[IBIS ver]   4.2
[File name]   msp432e411ytzad_212bga_v0p0.ibs
[File Rev]   v0p0
[Date]   Oct 10, 2017
[Source]   simulation
[Notes]   IBIS models for 212BGA package with updated GPIO models
[Disclaimer] Please be aware that in the absence of a written agreement,
   Texas Instruments (TI) assumes no liability for: 1) the
   accuracy of the IBIS models provided to your company, 2) the
   proper functioning of these IBIS models in your design or for
   any resulting applications, or; 3) infringement of patents,
   copyrights, or intellectual property rights resulting from
   your use of these IBIS models. TI provides IBIS models as a
   service to our customers and therefore reserves the right to
   limit distribution of the IBIS models.
   This preliminary model does not contain all of the possible pad
   models for each of the pad types.  The most commonly used modes
   have been provided and the next update will include all of the
   pad model combinations.
   The only missing models that needs to be highlighted are the
   model for the USB D+ and D- GPIOs and the Ethernet PHY.
   Currently only the USB functionality is provided on the D+ and
   D- pins.  Customers needing to model the PGIOs associated with
   these pins should check for a newer model.  The Ethernet pins
   are curently shown as NC.  Although models will be provided in
   a future release, the magnetics and connector should be palced
   as close as possible to the device for best performance.
[Copyright]   Property of Texas Instruments Incorporated. Unauthorized
   reproduction and/or distribution is strictly prohibited. This
   product is protected under copyright law and trade secret law
   as an unpublished work. Copyright (C) 2017, Texas Instruments
   Incorporated, all rights reserved. These commodities are under
   the U.S. Government distribution license control. As such,
   they are not to be re-exported without the prior approval of
   the U.S. Department of Commerce.
|   Component MSP432E411YTZAD
[Component]   MSP432E411YTZAD
[Manufacturer]   Texas Instruments Inc.
[Package]
| 212-pin BGA
| variable   typ   min   max
R_Pkg   1.91E-01   1.42E-01   3.53E-01
L_pkg   2.25E-09   1.34E-09   5.30E-09
C_pkg   5.40E-13   3.57E-13   1.22E-12
[Pin]   signal_name   model_name   R_pin   L_pin   C_pin
A1   GND   GND
A2   GND   GND
A4   PD4   GPIO12P   2.07E-01   2.54212E-09   4.28804E-13
A5   PE4   GPIO12P   2.01E-01   2.46532E-09   4.18963E-13
A7   PE6   GPIO12P   1.94E-01   2.38893E-09   4.10699E-13
A8   PP7   GPIO12P   1.96E-01   2.49906E-09   4.59589E-13
A10   PN4   GPIO12P   1.93E-01   2.41012E-09   3.56985E-13
A11   PN2   GPIO12P   1.94E-01   2.32364E-09   3.86379E-13
A13   PQ4   GPIO12P   2.11E-01   2.54553E-09   4.60355E-13
A14   PS3   GPIO12P   2.08E-01   2.42399E-09   4.21739E-13
A16   PB0   GPIO8P_5V   2.00E-01   3.23551E-09   6.06843E-13
A17   PB2   GPIO12P   2.14E-01   3.52368E-09   5.43338E-13
A18   GND   GND
A19   GND   GND
B1   GND   GND
B2   PD7   GPIO12P   1.72E-01   2.14055E-09   4.66734E-13
B3   PD6   GPIO12P   1.60E-01   1.98098E-09   4.32256E-13
B4   PD5   GPIO12P   2.13E-01   2.5073E-09   4.43666E-13
B5   PE5   GPIO12P   1.84E-01   2.03073E-09   4.37429E-13
B6   PB5   GPIO12P   1.58E-01   1.89444E-09   4.1673E-13
B7   PE7   GPIO12P   1.80E-01   1.97736E-09   4.23857E-13
B8   PP6   GPIO12P   1.90E-01   2.22432E-09   5.22651E-13
B9   PN5   GPIO12P   1.82E-01   2.16136E-09   4.15561E-13
B10   PN3   GPIO12P   1.77E-01   1.88683E-09   4.78218E-13
B11   PN1   GPIO12P   1.91E-01   2.18653E-09   4.34655E-13
B12   PP5   GPIO12P   1.86E-01   2.07672E-09   4.02153E-13
B13   PP2   GPIO12P   1.89E-01   2.06075E-09   4.92489E-13
B14   PS2   GPIO12P   1.99E-01   2.10108E-09   5.561E-13
B15   PC0_TCK_SWCL  GPIO12P   1.68E-01   1.94142E-09   4.56132E-13
B16   PB1   GPIO8P_5V   1.81E-01   2.72841E-09   5.97666E-13
B17   PB3   GPIO12P   1.72E-01   2.78265E-09   5.99724E-13
B18   PL7   USB_PHY_DM   2.19E-01   3.04557E-09   5.12885E-13
B19   GND   GND
C1   PD1   GPIO12P   2.23E-01   2.4804E-09   4.48859E-13
C2   PD0   GPIO12P   2.20E-01   2.41682E-09   4.37382E-13
C5   NC   NC
C6   PB4   GPIO12P   1.46E-01   1.54912E-09   4.45802E-13
C8   PJ0   GPIO2   1.80E-01   1.82529E-09   4.83027E-13
C10   PN0   GPIO12P   1.84E-01   1.89386E-09   4.95972E-13
C12   PP3   GPIO12P   1.87E-01   1.91608E-09   5.35179E-13
C14   PC3_TDO_SWO   GPIO12P   1.61E-01   1.74925E-09   6.28695E-13
C15   PC1_TMS_SWDIO GPIO12P   1.48E-01   1.52934E-09   4.82116E-13
C18   PL6   USB_PHY_DP   2.07E-01   2.63628E-09   4.79427E-13
D1   PD3   GPIO12P   2.09E-01   2.39664E-09   4.32E-13
D2   PD2   GPIO12P   1.98E-01   2.02977E-09   4.63339E-13
D6   PP0   GPIO12P   1.58E-01   1.68527E-09   6.86711E-13
D7   PP1   GPIO12P   1.42E-01   1.35133E-09   5.40685E-13
D8   PP4   GPIO12P   2.32E-01   2.94869E-09   9.1381E-13
D12   PS0   GPIO12P   2.22E-01   2.48323E-09   6.86306E-13
D13   PS1   GPIO12P   1.98E-01   2.00652E-09   5.4804E-13
D14   PC2_TDI   GPIO12P   1.53E-01   1.54259E-09   6.34879E-13
D18   GNDX2   GND
D19   OSC1   NC
E2   PQ1   GPIO12P   1.84E-01   1.9309E-09   4.33284E-13
E3   PQ0   GPIO12P   1.90E-01   1.89165E-09   5.26905E-13
E7   PJ1   GPIO2   1.98E-01   2.02835E-09   6.19666E-13
E10   VDDC   POWER
E13   NC   NC
E17   PJ5   GPIO12P   2.17E-01   3.0538E-09   6.50619E-13
E18   PT2   GPIO12P   2.17E-01   2.847E-09   6.05007E-13
E19   OSC0   NC
F1   PB7   GPIO12P   2.02E-01   2.45336E-09   4.57478E-13
F2   PB6   GPIO12P   1.83E-01   1.96383E-09   4.71815E-13
F3   VDDA   POWER
F4   VREFAP   NC
F10   GND   GND
F16   PJ3   GPIO12P   1.83E-01   2.23051E-09   7.29941E-13
F17   PT3   GPIO12P   1.83E-01   2.10068E-09   5.99792E-13
F18   PJ4   GPIO12P   2.06E-01   2.70644E-09   5.81715E-13
G1   PE2   GPIO12P   1.96E-01   2.36013E-09   4.29657E-13
G2   PE3   GPIO12P   1.94E-01   2.21348E-09   5.06269E-13
G4   GNDA   GND
G5   VREFAM   NC
G10   VDD   POWER
G15   PM5   GPIO8P   2.71E-01   3.62889E-09   9.78927E-13
G16   PL0   GPIO12P   1.60E-01   2.05833E-09   6.9482E-13
G18   PL2   GPIO12P   2.12E-01   2.9588E-09   6.34002E-13
G19   PL5   GPIO12P   1.89E-01   2.58913E-09   4.9052E-13
H2   PE1   GPIO12P   1.80E-01   1.87494E-09   4.25958E-13
H3   PE0   GPIO12P   1.77E-01   1.73654E-09   4.49528E-13
H4   PQ2   GPIO12P   2.11E-01   2.11091E-09   7.20307E-13
H9   VDD   POWER
H10   GND   GND
H11   GND   GND
H12   GND   GND
H16   VDDC   POWER
H17   PJ2   GPIO12P   1.56E-01   1.55215E-09   4.7763E-13
H18   PL4   GPIO12P   1.72E-01   2.02913E-09   5.32926E-13
H19   PL1   GPIO12P   1.92E-01   2.5474E-09   5.41353E-13
J1   PK0   GPIO12P   1.77E-01   2.02149E-09   4.06553E-13
J2   PK1   GPIO12P   1.74E-01   1.72918E-09   4.59484E-13
J8   VDD   POWER
J9   VDD   POWER
J10   VDD   POWER
J11   GND   GND
J12   GND   GND
J18   PL3   GPIO12P   1.66E-01   1.78848E-09   4.9918E-13
K1   PK2   GPIO12P   1.92E-01   2.27762E-09   4.57169E-13
K2   PK3   GPIO12P   1.73E-01   1.80579E-09   4.73887E-13
K3   PC7   GPIO12P   1.86E-01   1.81643E-09   5.0489E-13
K5   PJ7   GPIO12P   1.89E-01   1.8865E-09   6.38258E-13
K6   GND   GND
K7   VDD   POWER
K8   VDD   POWER
K9   GND   GND
K10   GND   GND
K11   VDD   POWER
K12   VDD   POWER
K13   GND   GND
K14   GND   GND
K15   PG5   GPIO12P   2.98E-01   4.06442E-09   1.19088E-12
K17   PG4   GPIO12P   3.53E-01   5.30125E-09   1.22467E-12
K18   PM0   GPIO12P   1.59E-01   1.82119E-09   4.71844E-13
K19   PM1   GPIO12P   1.81E-01   2.28041E-09   4.70777E-13
L2   PC6   GPIO12P   1.79E-01   1.84691E-09   4.4981E-13
L8   GND   GND
L9   GND   GND
L10   VDD   POWER
L11   VDD   POWER
L12   VDD   POWER
L18   PM2   GPIO12P   1.58E-01   1.7333E-09   4.53333E-13
L19   PM3   GPIO12P   1.74E-01   2.16602E-09   4.19113E-13
M1   PC5   GPIO12P   1.99E-01   2.43507E-09   4.10363E-13
M2   PC4   GPIO12P   1.96E-01   2.21573E-09   4.88755E-13
M3   PQ7   GPIO12P   1.81E-01   1.79585E-09   5.10188E-13
M4   PQ3   GPIO12P   2.07E-01   2.1296E-09   6.72323E-13
M8   GND   GND
M9   GND   GND
M10   GND   GND
M11   VDD   POWER
M12   VDD   POWER
M16   PG3   GPIO12P   2.80E-01   4.14075E-09   1.09773E-12
M17   HIB_n   HIB_OUTPUT   1.96E-01   2.45363E-09   7.43635E-13
M18   PM4   GPIO8P   1.61E-01   1.80256E-09   4.52048E-13
N1   PJ6   GPIO12P   1.95E-01   2.37484E-09   4.41642E-13
N2   PR2   GPIO12P   1.75E-01   1.73711E-09   4.72744E-13
N4   PR1   GPIO12P   1.91E-01   1.93106E-09   5.63332E-13
N5   PR0   GPIO12P   2.17E-01   2.28531E-09   6.69802E-13
N10   GND   GND
N15   PG0   GPIO12P   2.93E-01   3.93152E-09   1.06666E-12
N16   VDD   POWER
N18   PM7   GPIO8P   1.64E-01   1.6113E-09   4.65699E-13
N19   PM6   GPIO8P   1.66E-01   1.97917E-09   4.12294E-13
P2   PR5   GPIO12P   1.94E-01   2.13402E-09   4.7551E-13
P3   PR4   GPIO12P   1.95E-01   2.1522E-09   5.47923E-13
P4   PH0   GPIO12P   1.44E-01   1.34362E-09   5.35433E-13
P10   VDD   POWER
P16   GND   GND
P17   VDD   POWER
P18   RST_n   RST_INPUT   1.68E-01   1.91162E-09   4.3764E-13
P19   VBAT   POWER
R1   PH2   GPIO12P   2.00E-01   2.23416E-09   4.28776E-13
R2   PH1   GPIO12P   1.83E-01   1.77877E-09   4.53688E-13
R3   PH4   GPIO12P   1.51E-01   1.47303E-09   4.25059E-13
R7   PA7   GPIO12P   1.46E-01   1.41333E-09   6.01859E-13
R10   PR7   GPIO12P   1.45E-01   1.53519E-09   6.87491E-13
R13   PS7   GPIO12P   1.80E-01   2.55118E-09   1.08108E-12
R17   GND   GND
R18   GNDX   GND
T1   PH3   GPIO12P   2.06E-01   2.32889E-09   4.06305E-13
T2   PH5   GPIO12P   2.16E-01   2.41322E-09   5.00559E-13
T6   PA2   GPIO12P   1.56E-01   1.65304E-09   6.66079E-13
T7   PF3   GPIO12P   1.91E-01   1.87011E-09   5.55265E-13
T8   PF6   GPIO12P   1.98E-01   1.98922E-09   6.4558E-13
T12   PN6   GPIO12P   1.67E-01   1.93412E-09   6.62062E-13
T13   PS5   GPIO12P   1.79E-01   2.67893E-09   8.4824E-13
T14   PG1   GPIO12P   2.03E-01   2.73254E-09   8.27959E-13
T18   XOSC0   NC
T19   XOSC1   NC
U2   PH6   GPIO12P   2.13E-01   2.36723E-09   5.03622E-13
U5   PA3   GPIO12P   1.48E-01   1.57272E-09   4.95301E-13
U6   PF0   GPIO12P   1.98E-01   1.95399E-09   5.26644E-13
U8   PF7   GPIO12P   1.76E-01   1.74098E-09   5.24907E-13
U10   PS6   GPIO12P   1.77E-01   1.88304E-09   4.91443E-13
U12   PN7   GPIO12P   2.36E-01   3.14272E-09   6.59593E-13
U14   PG7   GPIO12P   1.78E-01   2.28069E-09   6.39138E-13
U15   PQ6   GPIO12P   2.14E-01   2.81733E-09   6.67747E-13
U18   WAKE_n   WAKE_INPUT   1.52E-01   2.11442E-09   3.7503E-13
U19   PK4   GPIO12P   2.02E-01   3.05079E-09   4.9169E-13
V1   GND   GND
V2   PH7   GPIO12P   2.10E-01   2.36221E-09   4.83971E-13
V3   PA0   GPIO12P   1.83E-01   2.22762E-09   4.48301E-13
V4   PA4   GPIO12P   1.99E-01   2.11561E-09   4.44869E-13
V5   PA6   GPIO12P   1.94E-01   2.10283E-09   4.37703E-13
V6   PF1   GPIO12P   1.88E-01   2.03569E-09   4.78105E-13
V7   PF4   GPIO12P   1.86E-01   2.04076E-09   5.16472E-13
V8   PR3   GPIO12P   2.04E-01   2.32022E-09   5.39242E-13
V9   PS4   GPIO12P   1.90E-01   2.16803E-09   5.02279E-13
V10   PT1   GPIO12P   1.79E-01   2.0276E-09   4.7391E-13
V11   PG2   GPIO12P   1.75E-01   1.94098E-09   4.53654E-13
V12   PG6   GPIO12P   1.80E-01   1.9975E-09   4.76869E-13
V13   EN0RXIN   NC
V14   EN0TXON   NC
V15   EN0TXOP   NC
V16   PK6   GPIO12P   1.84E-01   2.27053E-09   4.79628E-13
V17   PK5   GPIO12P   1.89E-01   2.54531E-09   4.72275E-13
V18   NC   NC
V19   NC   NC
W1   GND   GND
W2   GND   GND
W3   PA1   GPIO12P   2.02E-01   2.58768E-09   5.06478E-13
W4   PA5   GPIO12P   2.19E-01   2.54645E-09   4.45583E-13
W6   PF2   GPIO12P   1.91E-01   2.4123E-09   4.85889E-13
W7   PF5   GPIO12P   2.05E-01   2.44149E-09   5.01309E-13
W9   PR6   GPIO12P   1.97E-01   2.47666E-09   5.02948E-13
W10   PT0   GPIO12P   2.01E-01   2.46772E-09   4.90488E-13
W12   PQ5   GPIO12P   2.00E-01   2.44147E-09   4.56967E-13
W13   EN0RXIP   NC
W15   RBIAS   NC
W16   PK7   GPIO12P   1.92E-01   2.60076E-09   4.41066E-13
W18   NC   NC
W19   NC   NC
[Model Selector] GPIO12P
GPIO12P_I/O_2   2mA Output Buffer
GPIO12P_I/O_4   4mA Output Buffer
GPIO12P_I/O_8S   8mA Output Buffer with Slew Rate Control
GPIO12P_I/O_8   8mA Output Buffer
GPIO12P_I/O_12S   12mA Output Buffer with Slew Rate Control
GPIO12P_I/O_12   12mA Output Buffer
GPIO12P_I_WPU_2   2ma Input with Pull-Up
GPIO12P_I_WPD_2   2mA Input with Pull-Down
GPIO12P_I/O_OD_2   2mA Output Buffer with Open Drain
GPIO12P_I/O_OD_4   4mA Output Buffer with Open Drain
GPIO12P_I/O_OD_8S   8mA Output Buffer with Open Drain and Slew Rate Control
GPIO12P_I/O_OD_8   8mA Output Buffer with Open Drain
GPIO12P_I/O_OD_12S   12mA Output Buffer with Open Drain and Slew Rate Control
GPIO12P_I/O_OD_12   12mA Output Buffer with Open Drain
[Model Selector] GPIO8P
GPIO8P_I/O_2   2mA Output Buffer
GPIO8P_I/O_4   4mA Output Buffer
GPIO8P_I/O_8S   8mA Output Buffer with Slew Rate Control
GPIO8P_I/O_8   8mA Output Buffer
GPIO8P_I_WPU_2   2mA Input with Pull-Up
GPIO8P_I_WPD_2   2mA Input with Pull-Down
GPIO8P_I/O_OD_2   2mA Output Buffer with Open Drain
GPIO8P_I/O_OD_4   4mA Output Buffer with Open Drain
GPIO8P_I/O_OD_8S   8mA Output Buffer with Open Drain and Slew Rate Control
GPIO8P_I/O_OD_8   8mA Output Buffer with Open Drain
GPIO8P_I_TAMPER   Tamper Input Model
GPIO8P_I_TAMPER_VWPU   Tamper Input Model with Very Weak Pull-Up
[Model Selector] GPIO8P_5V
GPIO8P_5V_I/O_2   2mA Output Buffer
GPIO8P_5V_I/O_4   4mA Output Buffer
GPIO8P_5V_I/O_8S   8mA Output Buffer with Slew Rate Control
GPIO8P_5V_I/O_8   8mA Output Buffer
GPIO8P_5V_I_WPU_2   2mA Input with Pull-Up
GPIO8P_5V_I_WPD_2   2mA Input with Pull-Down
GPIO8P_5V_I/O_OD_2   2mA Output Buffer with Open Drain
GPIO8P_5V_I/O_OD_4   4mA Output Buffer with Open Drain
GPIO8P_5V_I/O_OD_8S   8mA Output Buffer with Open Drain and Slew Rate Control
GPIO8P_5V_I/O_OD_8   8mA Output Buffer with Open Drain
[Model Selector] GPIO2
GPIO2_I/O_2   2mA Output Buffer
GPIO2_I_WPU_2   2mA Input with Pull-Up
GPIO2_I_WPD_2   2mA Input with Pull-Down
GPIO2_I/O_OD_2   GPIO2_I/O_OD_2
[Model Selector] RST_INPUT
RESET_INPUT   Reset Pad Input Model
[Model Selector] HIB_OUTPUT
HIBERNATE_OUTPUT   Output Buffer for the HIB_n Pin
[Model Selector] WAKE_INPUT
WAKE_IN   Input Model for the WAKE_n Pin
[Model Selector] USB_PHY_DP
fsdp_tx   Full Speed transmitter--12Mbps
lsdp_50pf_tx   Low speed transmitter--1.5Mbps driving 50pF cap load
lsdp_200pf_tx   Low speed transmitter--1.5Mbps driving 200pF cap load
lsdp_400pf_tx   Low speed transmitter--1.5Mbps driving 400pF cap load
lsdp_600pf_tx   Low speed transmitter--1.5Mbps driving 600pF cap load
fsdp_rx   Recieve mode--Open circuit during fs/ls recieve mode
[Model Selector] USB_PHY_DM
fsdm_tx   Full Speed transmitter--12Mbps
lsdm_50pf_tx   Low speed transmitter--1.5Mbps driving 50pF cap load
lsdm_200pf_tx   Low speed transmitter--1.5Mbps driving 200pF cap load
lsdm_400pf_tx   Low speed transmitter--1.5Mbps driving 400pF cap load
lsdm_600pf_tx 	 Low speed transmitter--1.5Mbps driving 600pF cap load
fsdm_rx   Recieve mode--Open circuit during fs/ls recieve mode
| Models and submodels in the file (55): GPIO12P_I/O_2 (I/O), GPIO12P_I/O_4 (I/O), GPIO12P_I/O_8S (I/O), GPIO12P_I/O_8 (I/O), GPIO12P_I/O_12S (I/O), GPIO12P_I/O_12 (I/O), GPIO12P_I_WPU_2 (Input), GPIO12P_I_WPD_2 (Input), GPIO12P_I/O_OD_2 (I/O_open_drain), GPIO12P_I/O_OD_4 (I/O_open_drain), GPIO12P_I/O_OD_8S (I/O_open_drain), GPIO12P_I/O_OD_8 (I/O_open_drain), GPIO12P_I/O_OD_12S (I/O_open_drain), GPIO12P_I/O_OD_12 (I/O_open_drain), GPIO8P_I/O_2 (I/O), GPIO8P_I/O_4 (I/O), GPIO8P_I/O_8S (I/O), GPIO8P_I/O_8 (I/O), GPIO8P_I_WPU_2 (Input), GPIO8P_I_WPD_2 (Input), GPIO8P_I/O_OD_2 (I/O_open_drain), GPIO8P_I/O_OD_4 (I/O_open_drain), GPIO8P_I/O_OD_8S (I/O_open_drain), GPIO8P_I/O_OD_8 (I/O_open_drain), GPIO8P_I_TAMPER (Input), GPIO8P_I_TAMPER_VWPU (Input), GPIO8P_5V_I/O_2 (I/O), GPIO8P_5V_I/O_4 (I/O), GPIO8P_5V_I/O_8S (I/O), GPIO8P_5V_I/O_8 (I/O), GPIO8P_5V_I_WPU_2 (Input), GPIO8P_5V_I_WPD_2 (Input), GPIO8P_5V_I/O_OD_2 (I/O_open_drain), GPIO8P_5V_I/O_OD_4 (I/O_open_drain), GPIO8P_5V_I/O_OD_8S (I/O_open_drain), GPIO8P_5V_I/O_OD_8 (I/O_open_drain), GPIO2_I/O_2 (I/O), GPIO2_I_WPU_2 (Input), GPIO2_I_WPD_2 (Input), GPIO2_I/O_OD_2 (I/O_open_drain), RESET_INPUT (Input), HIBERNATE_OUTPUT (Output), WAKE_IN (Input), fsdp_tx (3-state), lsdp_50pf_tx (3-state), lsdp_200pf_tx (3-state), lsdp_400pf_tx (3-state), lsdp_600pf_tx (3-state), fsdp_rx (Input), fsdm_tx (3-state), lsdm_50pf_tx (3-state), lsdm_200pf_tx (3-state), lsdm_400pf_tx (3-state), lsdm_600pf_tx (3-state), fsdm_rx (Input)
